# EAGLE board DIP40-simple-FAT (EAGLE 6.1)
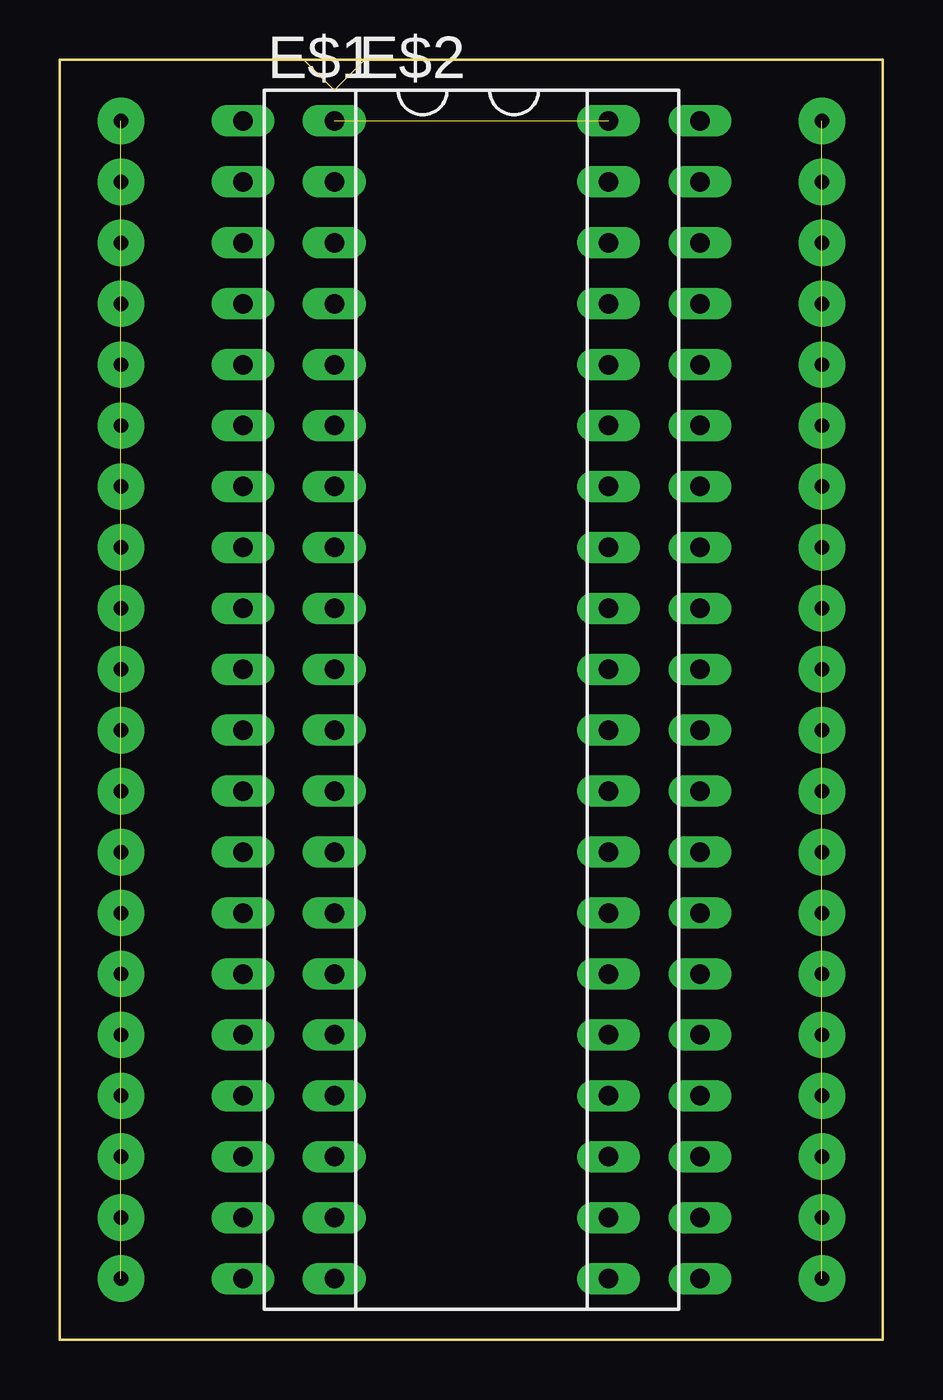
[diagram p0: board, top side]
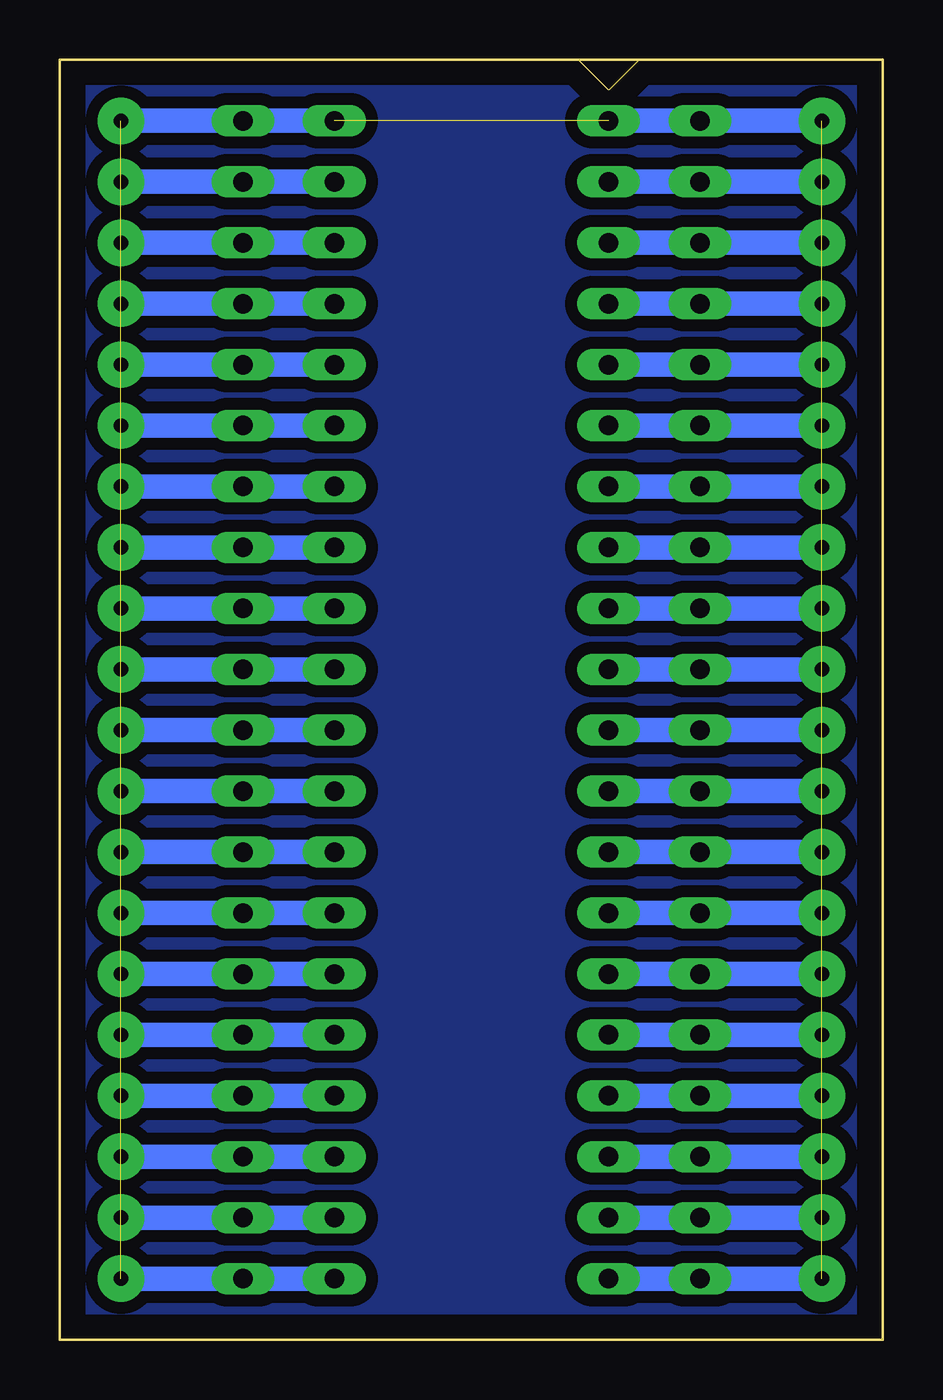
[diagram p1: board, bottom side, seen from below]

Size 34.29 x 53.34 mm. Coordinates in mm from the lower left corner, seen from the top.
Outline: 0,53.34 34.29,53.34 34.29,0 0,0 0,53.34
Copper layers (1*16): Top 0.035mm / dielectric 1.5mm / Bottom 0.035mm
Design rules: minimum track width 10mil, minimum drill 24mil, track to track 8mil, track to pad 8mil, pad to pad 8mil, via to via 8mil, smd to smd 8mil, copper to edge 40mil, drill to drill 8mil, minimum pad ring 10mil, minimum via ring 8mil, stop-mask expansion 4mil, vias tented up to drill 0mil, thermal gap 10mil

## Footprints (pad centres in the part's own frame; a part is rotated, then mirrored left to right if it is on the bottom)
DIL40 = drill 0.813 long: 1 -24.13,-7.62; 2 -21.59,-7.62; 3 -19.05,-7.62; 4 -16.51,-7.62; 5 -13.97,-7.62; 6 -11.43,-7.62; 7 -8.89,-7.62; 8 -6.35,-7.62; 9 -3.81,-7.62; 10 -1.27,-7.62; 11 1.27,-7.62; 12 3.81,-7.62; 13 6.35,-7.62; 14 8.89,-7.62; 15 11.43,-7.62; 16 13.97,-7.62; 17 16.51,-7.62; 18 19.05,-7.62; 19 21.59,-7.62; 20 24.13,-7.62; 21 24.13,7.62; 22 21.59,7.62; 23 19.05,7.62; 24 16.51,7.62; 25 13.97,7.62; 26 11.43,7.62; 27 8.89,7.62; 28 6.35,7.62; 29 3.81,7.62; 30 1.27,7.62; 31 -1.27,7.62; 32 -3.81,7.62; 33 -6.35,7.62; 34 -8.89,7.62; 35 -11.43,7.62; 36 -13.97,7.62; 37 -16.51,7.62; 38 -19.05,7.62; 39 -21.59,7.62; 40 -24.13,7.62

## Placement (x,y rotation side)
E$1  [DIL40]  15.24,26.67 270 top
E$2  [DIL40]  19.05,26.67 270 top

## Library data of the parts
E$1 E$2 = 74xx-us

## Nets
S$2: E$2.1

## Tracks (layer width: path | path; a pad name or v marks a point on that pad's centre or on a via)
S$2  (via drill 0.6 pad 1.93)  (39 unrouted)
  Bottom 0.406: v2.54,50.8 E$2.1 | v2.54,48.26 11.43,48.26 | v2.54,45.72 11.43,45.72 | v2.54,43.18 11.43,43.18 | v2.54,40.64 11.43,40.64 | v2.54,38.1 11.43,38.1 | v2.54,33.02 11.43,33.02 | v2.54,30.48 11.43,30.48 | v2.54,27.94 11.43,27.94 | v2.54,25.4 11.43,25.4 | v2.54,22.86 11.43,22.86 | v2.54,20.32 11.43,20.32 | v2.54,17.78 11.43,17.78 | v2.54,15.24 11.43,15.24 | v2.54,12.7 11.43,12.7 | v2.54,10.16 11.43,10.16 | v2.54,7.62 11.43,7.62 | v2.54,5.08 11.43,5.08 | v2.54,2.54 11.43,2.54
  Bottom 1.016: v2.54,35.56 11.43,35.56 | v2.54,38.1 11.43,38.1 | v2.54,40.64 11.43,40.64 | v2.54,43.18 11.43,43.18 | v2.54,45.72 11.43,45.72 | v2.54,48.26 11.43,48.26 | v2.54,50.8 E$2.1 | v2.54,33.02 11.43,33.02 | v2.54,30.48 11.43,30.48 | v2.54,27.94 11.43,27.94 | v2.54,25.4 11.43,25.4 | v2.54,22.86 11.43,22.86 | v2.54,20.32 11.43,20.32 | v2.54,17.78 11.43,17.78 | v2.54,15.24 11.43,15.24 | v2.54,12.7 11.43,12.7 | v2.54,10.16 11.43,10.16 | v2.54,7.62 11.43,7.62 | v2.54,5.08 11.43,5.08 | v2.54,2.54 11.43,2.54 | 22.86,2.54 v31.75,2.54 | 22.86,5.08 v31.75,5.08 | 22.86,7.62 v31.75,7.62 | 22.86,10.16 v31.75,10.16 | 22.86,12.7 v31.75,12.7 | 22.86,15.24 v31.75,15.24 | 22.86,17.78 v31.75,17.78 | 22.86,20.32 v31.75,20.32 | 22.86,22.86 v31.75,22.86 | 22.86,25.4 v31.75,25.4 | 22.86,27.94 v31.75,27.94 | 22.86,30.48 v31.75,30.48 | 22.86,33.02 v31.75,33.02 | 22.86,35.56 v31.75,35.56 | 22.86,38.1 v31.75,38.1 | 22.86,40.64 v31.75,40.64 | 22.86,43.18 v31.75,43.18 | 22.86,45.72 v31.75,45.72 | 22.86,48.26 v31.75,48.26 | 22.86,50.8 v31.75,50.8
S$3  (via drill 0.6 pad 1.7)
  other vias: 2.54,48.26
S$4  (via drill 0.6 pad 1.7)  (1 unrouted)
  other vias: 2.54,50.8 2.54,50.8 2.54,50.8 2.54,48.26
S$22  (16 unrouted)
  Bottom 0.406: 31.75,2.54 22.86,2.54 | 31.75,5.08 22.86,5.08 | 31.75,7.62 22.86,7.62 | 31.75,10.16 22.86,10.16 | 31.75,12.7 22.86,12.7 | 31.75,15.24 22.86,15.24 | 31.75,17.78 22.86,17.78 | 31.75,20.32 22.86,20.32 | 31.75,22.86 22.86,22.86 | 31.75,25.4 22.86,25.4 | 31.75,27.94 22.86,27.94 | 31.75,30.48 22.86,30.48 | 31.75,35.56 22.86,35.56 | 31.75,40.64 22.86,40.64 | 31.75,45.72 22.86,45.72 | 31.75,48.26 22.86,48.26 | 31.75,50.8 22.86,50.8
S$41
  pour Bottom (isolate 0.5): 0,53.34 34.29,53.34 34.29,0 0,0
